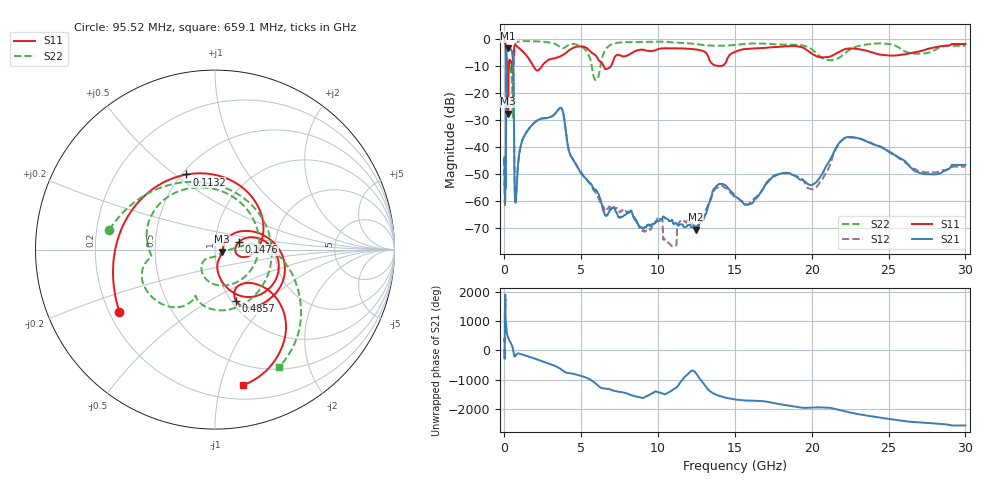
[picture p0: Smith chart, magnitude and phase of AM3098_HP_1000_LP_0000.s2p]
! Date/Time: Thu, Feb 28, 2019 8:39 AM
! Network Analyzer: Agilent Technologies E8364B Rev: A.07.50.67
! Sweep from 0.010 to 30.000 GHz, 1601 Points, Sweep Type: LOG
! Power Supply: 5.023 V, 0.002 A
# Hz S DB R 50
!freq MagS11 AngS11 MagS21 AngS21 MagS12 AngS12 MagS22 AngS22
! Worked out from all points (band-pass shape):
!   1601 points, 10 MHz to 30 GHz, reference 50 ohm
!   highest |S21| = -3.24 dB at 235.1 MHz (marker M1); lowest = -70.8 dB at 12.43 GHz (marker M2)
!   |S21| within 3 dB of the highest: 127.3 MHz to 537.8 MHz (410.5 MHz wide, 123 % of centre)
!   lowest |S11| = -27.6 dB at 237.5 MHz (marker M3), VSWR 1.09, Z = 54.2 - j1.22 ohm
!   |S11| at or under -10 dB: 198.3 MHz to 290.8 MHz (92.59 MHz wide, 37.9 % of centre); 1.889 GHz to 2.425 GHz (536.4 MHz wide, 24.9 % of centre); 6.475 GHz to 6.923 GHz (448.3 MHz wide, 6.69 % of centre)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
!   |S22| runs from -29.0 to -0.5 dB; largest |S21 - S12| = 0.012
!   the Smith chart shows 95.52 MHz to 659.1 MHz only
!   S11 on the Smith chart (normalised r, x): 95.52 MHz: 0.24, -0.28; 113.2 MHz: 0.53, +0.55; 147.6 MHz: 1.30, +0.11; 485.7 MHz: 1.05, -0.67; 659.1 MHz: 0.31, -1.17
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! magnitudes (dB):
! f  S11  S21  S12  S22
! 10 MHz  -0.4  -45.5  -44.4  -0.5
! 38.04 MHz  -0.5  -60.2  -61.6  -0.7
! 95.52 MHz  -3.9  -42.4  -42.5  -4.5
! 113.2 MHz  -7.0  -15.7  -15.7  -10.1
! 144.7 MHz  -18.4  -4.2  -4.2  -10.4
! 147.6 MHz  -17.1  -4.1  -4.1  -9.9
! 190.6 MHz  -9.0  -3.7  -3.7  -7.2
! 235.1 MHz  -27.4  -3.2  -3.2  -9.0
! 237.5 MHz  -27.6  -3.2  -3.2  -9.0
! 302 MHz  -9.0  -3.5  -3.4  -7.9
! 485.7 MHz  -10.1  -4.4  -4.4  -15.4
! 550.5 MHz  -11.2  -7.2  -7.2  -27.4
! 659.1 MHz  -2.2  -53.9  -53.3  -2.5
! 728.5 MHz  -2.1  -59.8  -60.3  -1.3
! 2.084 GHz  -11.5  -30.3  -30.3  -0.7
! 3.686 GHz  -6.1  -25.5  -25.5  -3.1
! 5.959 GHz  -6.0  -56.0  -57.2  -15.2
! 7.926 GHz  -6.1  -65.0  -64.1  -1.0
! 12.43 GHz  -3.7  -70.8  -69.2  -1.7
! 20.2 GHz  -5.9  -53.4  -55.3  -4.6
! 22.56 GHz  -3.3  -36.3  -36.5  -3.5
! 30 GHz  -1.7  -46.7  -47.3  -2.4
